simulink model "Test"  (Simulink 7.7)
settings: Solver=VariableStepDiscrete  StartTime=0.0  StopTime=inf  MaxStep=0.05  RelTol=1e-3
PostLoadFcn:
  | Init_Arduino;
libraries: arduino_io_lib x5, simulink x2

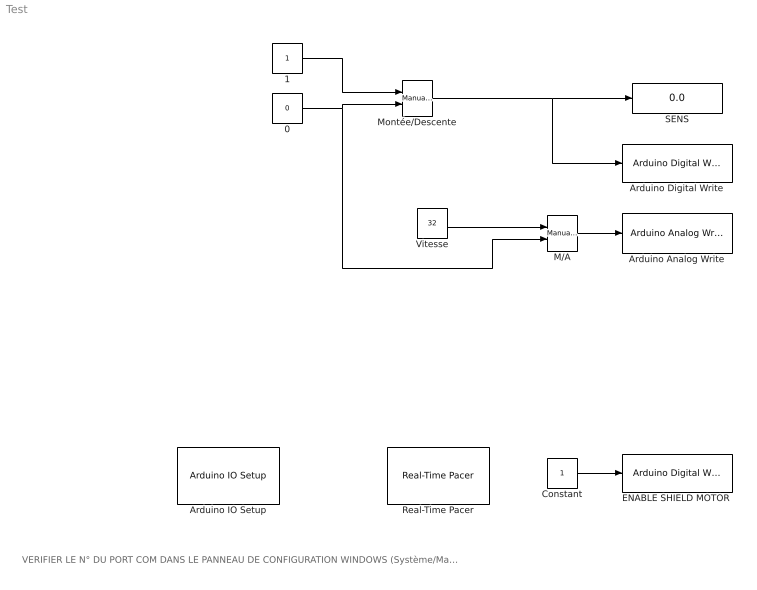
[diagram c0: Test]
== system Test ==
  note: VERIFIER LE N° DU PORT COM DANS LE PANNEAU DE CONFIGURATION WINDOWS (Système/Matériel/Gestionnaire de périphériques/Ports (COM et LPT))
  0 : Constant  Value=0
  1 : Constant
  Arduino Analog Write : arduino_io_lib/Arduino Analog Write  arduinoVar=Temporary arduino variable: Arduino1  arduinoPin=9  T=0.2
  Arduino Digital Write : arduino_io_lib/Arduino Digital Write  arduinoVar=Temporary arduino variable: Arduino1  arduinoPin=7  T=0.2
  Arduino IO Setup : arduino_io_lib/Arduino IO Setup  Priority=3  arduinoVar=Temporary arduino variable: Arduino1  workspaceVarName=a  comPort=COM5
  Constant : Constant
  "ENABLE SHIELD MOTOR " : arduino_io_lib/Arduino Digital Write  arduinoVar=Temporary arduino variable: Arduino1  arduinoPin=4  T=0.2
  M/A : simulink/Signal Routing/Manual Switch  SystemSampleTime=-1  sw=0  action=0  varsize=off
  Montée/Descente : simulink/Signal Routing/Manual Switch  SystemSampleTime=-1  sw=1  action=0  varsize=off
  Real-Time Pacer : arduino_io_lib/Real-Time Pacer  simTimePerRealTime=.5
  SENS : Display
  Vitesse : Constant  Value=32
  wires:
  Constant/1 -> "ENABLE SHIELD MOTOR "/1
  0/1 -> Montée/Descente/2, M/A/2
  1/1 -> Montée/Descente/1
  M/A/1 -> Arduino Analog Write/1
  Vitesse/1 -> M/A/1
  Montée/Descente/1 -> SENS/1, Arduino Digital Write/1
